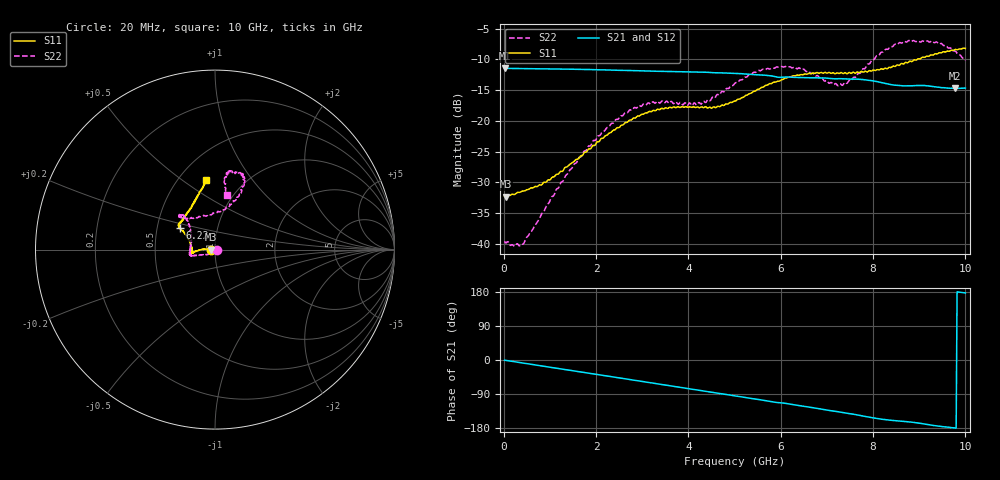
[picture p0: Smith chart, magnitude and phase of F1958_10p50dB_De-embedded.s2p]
! Integrated Device Technology
! Corporate Headquarters
! 6024 Silver Creek Valley Road
! San Jose, CA 95138  USA
! Phone:  1-408-284-8200
! Toll Free:  1-800-223-1366
! Webpage:  http://www.idt.com/
! Timing and RF Division
! 515 Groton Road, Suite 102
! Westford, MA 01886-6024
! Device:  F1958
! Description: 7-bit 0.25 dB Digital Step Attenuator
! Frequency:  0.001 -  6.000 GHz
! Package:  4x4 mm Thin QFN Plastic Package: 24 pin
! Ports:  2 RF, 12 DC
!  Pin  1  = D0
!  Pin  2  = VDD
!  Pin  3  = VMODE
!  Pin  4  = GND
!  Pin  5  = RF1  =  Port 1
!  Pin  6  = GND
!  Pin  7  = GND
!  Pin  8  = GND
!  Pin  9  = GND
!  Pin 10  = GND
!  Pin 11  = GND
!  Pin 12  = GND
!  Pin 13  = GND
!  Pin 14  = RF2  =  Port 2
!  Pin 15  = GND
!  Pin 16  = LE
!  Pin 17  = CLK
!  Pin 18  = DATA
!  Pin 19  = D6
!  Pin 20  = D5
!  Pin 21  = D4
!  Pin 22  = D3
!  Pin 23  = D2
!  Pin 24  = D1
! State:  42
! Atten State:  10.50 dB
! Voltage:  +3.30 Volts
! Current:  0.258 mA
! Data:  The device was measured on a F1958 evaluation board which has
!  individual transmission lines to the RF pins.  Data was collected
!  using a calibrated network analyzer.  The evaluation board was
!  de-embedded using Automatic Fixture Removal (AFR).
!  The reference plane is the edge of the package pin.
! Misc:
!  Action Tracker AT0419
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# GHz S dB R 50
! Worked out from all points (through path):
!   500 points, 20 MHz to 10 GHz, reference 50 ohm
!   highest |S21| = -11.43 dB at 20 MHz (marker M1); lowest = -14.7 dB at 9.78 GHz (marker M2)
!   group delay of S21, straight-line fit = 51.8 ps
!   lowest |S11| = -32.3 dB at 40 MHz (marker M3), VSWR 1.05, Z = 47.6 - j0.0732 ohm
!   |S11| at or under -10 dB: start of sweep to 8.954 GHz
!   |S22| runs from -40.4 to -6.9 dB; largest |S21 - S12| = 0.00093
!   S11 on the Smith chart (normalised r, x): 20 MHz: 0.95, -0.00; 6.22 GHz: 0.66, +0.16; 10 GHz: 0.67, +0.61
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0.02  -32.29 -178.3  -11.43 -0.5  -11.43 -0.5  -39.61 -10.5
0.04  -32.33 -178.2  -11.44 -0.9  -11.44 -0.9  -39.86 -16.8
0.42  -31.41 176.0  -11.49 -8.1  -11.49 -8.0  -40.07 -62.5
0.96  -29.60 176.0  -11.53 -18.2  -11.52 -18.2  -33.47 -113.6
1.7  -25.65 178.0  -11.62 -32.1  -11.62 -32.1  -25.52 -149.6
2.58  -20.66 -176.5  -11.77 -48.7  -11.76 -48.7  -19.15 -163.1
2.92  -19.19 -174.1  -11.83 -55.1  -11.82 -55.2  -17.54 -165.5
3.36  -18.15 -171.7  -11.93 -63.3  -11.93 -63.4  -17.00 -167.3
4.24  -17.87 -176.2  -12.06 -79.8  -12.07 -79.9  -17.02 165.2
4.64  -17.60 175.2  -12.17 -87.4  -12.18 -87.4  -15.69 147.5
5.02  -16.77 164.0  -12.26 -94.7  -12.27 -94.7  -13.78 136.1
5.54  -14.79 153.4  -12.51 -104.6  -12.52 -104.6  -11.81 133.2
6.22  -12.81 148.7  -12.88 -116.9  -12.89 -116.9  -11.25 137.4
6.68  -12.24 146.0  -12.98 -125.4  -13.00 -125.3  -12.26 132.7
7.1  -12.25 141.6  -13.10 -134.1  -13.11 -134.0  -13.75 115.5
7.36  -12.29 138.9  -13.15 -139.0  -13.16 -138.9  -14.01 93.9
7.9  -11.91 128.3  -13.37 -150.4  -13.37 -150.5  -10.72 69.6
8.34  -11.30 118.8  -14.02 -158.6  -14.02 -158.7  -8.21 65.6
8.74  -10.56 111.6  -14.30 -162.8  -14.31 -162.8  -7.12 69.2
9.24  -9.30 102.8  -14.36 -171.7  -14.37 -171.8  -7.14 78.3
9.78  -8.38 98.4  -14.71 -179.6  -14.74 -179.5  -8.63 81.1
10  -8.20 97.8  -14.65 176.9  -14.69 177.0  -10.16 77.2
